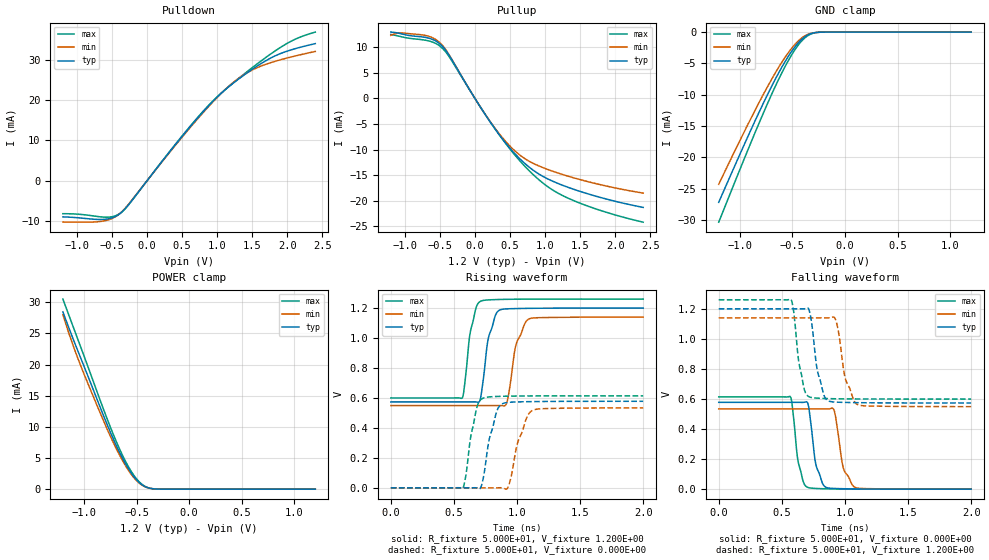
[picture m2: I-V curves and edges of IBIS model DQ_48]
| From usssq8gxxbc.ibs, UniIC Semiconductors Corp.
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|   Model DQ_48
[Model] DQ_48
Model_type I/O
Polarity   Non-Inverting
Enable   Active-High
Vinl =  8.300E-01
Vinh =  9.700E-01
Vmeas =  8.400E-01
Rref =  5.000E+01
Vref =  1.200E+00
C_comp   6.590E-13   6.530E-13   6.678E-13
C_comp_pullup   3.168E-13   3.162E-13   3.180E-13
C_comp_pulldown   3.268E-13   3.197E-13   3.362E-13
[Model Spec]
Vinh   9.700E-01   9.250E-01   1.015E+00
Vinl   8.300E-01   7.850E-01   8.750E-01
Vmeas   8.400E-01   7.980E-01   8.820E-01
Vref   1.200E+00   1.140E+00   1.260E+00
Rref   5.000E+01   5.000E+01   5.000E+01
[Temperature Range]   4.500E+01   9.500E+01   0.000E+00
[Voltage Range]   1.200E+00   1.140E+00   1.260E+00
[C Comp Corner]
C_comp_pullup   3.168E-13   3.180E-13   3.162E-13
C_comp_pulldown   3.268E-13   3.197E-13   3.362E-13
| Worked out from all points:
|   slope of the pulldown table from 0 to 0.18 V, typ, clamps not added: 44.6 ohm
|   slope of the pullup table from 0 to 0.18 V, typ, clamps not added: 46.9 ohm
|   GND clamp passes 1 mA (typ) near -0.40 V on its own axis
|   POWER clamp passes 1 mA (typ) near -0.47 V on its own axis
|   rising waveform, R_fixture 5.000E+01, V_fixture 1.200E+00: 20-80 % time 74.8ps typ, 87.1ps min, 65.1ps max; typ from 0.574 V to 1.2 V
|   rising waveform, R_fixture 5.000E+01, V_fixture 0.000E+00: 20-80 % time 80.7ps typ, 98.7ps min, 68.3ps max; typ from 0 V to 0.578 V
|   falling waveform, R_fixture 5.000E+01, V_fixture 0.000E+00: 20-80 % time 64.2ps typ, 69.4ps min, 57.5ps max; typ from 0.578 V to 0 V
|   falling waveform, R_fixture 5.000E+01, V_fixture 1.200E+00: 20-80 % time 70.3ps typ, 85.6ps min, 60.9ps max; typ from 1.2 V to 0.574 V
[Pulldown]
|Voltage   I(typ)   I(min)   I(max)
-1.2V     -8.95mA    -10.23mA   -8.16mA
-645mV    -9.589mA   -10.04mA   -8.974mA
-497mV    -9.184mA   -9.333mA   -8.904mA
-386mV    -8.143mA   -8.108mA   -8.086mA
-275mV    -6.168mA   -6.062mA   -6.22mA
687mV     14.86mA    14.65mA    15mA
983mV     20.46mA    20.34mA    20.53mA
1.205V    23.86mA    24.02mA    23.93mA
1.464V    27.19mA    27.13mA    27.55mA
1.797V    30.71mA    29.46mA    31.83mA
2.093V    32.65mA    30.85mA    34.92mA
2.4V      34mA       32.06mA    36.86mA
[Pullup]
|Voltage   I(typ)   I(min)   I(max)
-1.2V     12.95mA    12.32mA    12.49mA
-1.041V   12.59mA    12.78mA    12.02mA
-745mV    12mA       12.39mA    11.45mA
-486mV    10.48mA    10.69mA    10.06mA
-375mV    8.569mA    8.662mA    8.299mA
32mV      -704.1uA   -701.9uA   -692.2uA
291mV     -6.036mA   -5.916mA   -6.023mA
513mV     -9.935mA   -9.504mA   -10.11mA
735mV     -12.98mA   -11.95mA   -13.58mA
1.031V    -15.66mA   -13.83mA   -17.16mA
1.327V    -17.35mA   -15.18mA   -19.47mA
2.4V      -21.28mA   -18.49mA   -24.17mA
[GND_clamp]
|Voltage   I(typ)   I(min)   I(max)
-1.2V     -27.2mA    -24.33mA   -30.38mA
-875mV    -14.93mA   -13.17mA   -16.89mA
-750mV    -10.47mA   -9.157mA   -11.95mA
-650mV    -7.145mA   -6.184mA   -8.244mA
-575mV    -4.884mA   -4.175mA   -5.699mA
-500mV    -2.92mA    -2.45mA    -3.459mA
-425mV    -1.383mA   -1.13mA    -1.679mA
-375mV    -673.2uA   -542.8uA   -837uA
-300mV    -135.5uA   -116.3uA   -166.1uA
-225mV    -14.67uA   -15.93uA   -14.24uA
1.2V      0A         0A         0A
[POWER_clamp]
|Voltage   I(typ)   I(min)   I(max)
-1.2V     28.45mA    28mA       30.5mA
-1.125V   25.07mA    24.12mA    27.08mA
-1.025V   20.8mA     19.57mA    22.55mA
-850mV    13.34mA    12.42mA    14.46mA
-750mV    9.2mA      8.545mA    10.01mA
-650mV    5.523mA    5.115mA    6.037mA
-575mV    3.235mA    2.981mA    3.547mA
-500mV    1.501mA    1.371mA    1.657mA
-450mV    723.1uA    662.7uA    804.4uA
-375mV    148.3uA    148.7uA    156.1uA
-300mV    17.6uA     22.56uA    14.19uA
1.2V      0A         0A         0A
[Ramp]
| variable   typ   min   max
dV/dt_r   3.466E-01/8.120E-11   3.202E-01/9.979E-11   3.683E-01/6.823E-11
dV/dt_f   3.759E-01/7.046E-11   3.546E-01/8.551E-11   3.962E-01/6.107E-11
R_load = 5.000E+01
[Rising Waveform]
R_fixture= 5.000E+01
V_fixture= 1.200E+00
V_fixture_min= 1.140E+00
V_fixture_max= 1.260E+00
|time   V(typ)   V(min)   V(max)
0s        573.5mV    548.8mV    599.7mV
565ps     573.6mV    548.8mV    598.5mV
632ps     573.7mV    548.8mV    1.049V
712ps     603.2mV    548.9mV    1.246V
770ps     987.6mV    548.9mV    1.254V
856ps     1.184V     549.2mV    1.257V
916ps     1.194V     561.6mV    1.258V
986ps     1.196V     934.4mV    1.259V
1.086ns   1.198V     1.123V     1.259V
2ns       1.2V       1.14V      1.26V
[Rising Waveform]
R_fixture= 5.000E+01
V_fixture= 0.000E+00
V_fixture_min= 0.000E+00
V_fixture_max= 0.000E+00
|time   V(typ)   V(min)   V(max)
0s        212nV      624.9nV    103.2nV
571ps     74.47uV    23.77uV    -2.692mV
677ps     -125.2uV   66.44uV    521mV
740ps     99.55mV    55.33uV    601.2mV
788ps     351.8mV    73.19uV    607.5mV
884ps     561.1mV    -314.5uV   611mV
934ps     570.6mV    14.74mV    611.9mV
1.005ns   573.5mV    301.9mV    612.7mV
1.115ns   575.4mV    513.1mV    613.4mV
2ns       577.6mV    533.7mV    613.8mV
[Falling Waveform]
R_fixture= 5.000E+01
V_fixture= 0.000E+00
V_fixture_min= 0.000E+00
V_fixture_max= 0.000E+00
|time   V(typ)   V(min)   V(max)
0s        577.7mV    533.9mV    613.8mV
565ps     577.6mV    533.9mV    617.4mV
632ps     577.6mV    533.9mV    172.4mV
705ps     573.2mV    533.9mV    11.81mV
770ps     163.5mV    533.9mV    4.705mV
846ps     14.02mV    533.5mV    2.506mV
916ps     4.591mV    520.9mV    1.432mV
987ps     2.974mV    141.6mV    820uV
1.078ns   1.762mV    12.84mV    406.4uV
2ns       13.41uV    118.4uV    1.177uV
[Falling Waveform]
R_fixture= 5.000E+01
V_fixture= 1.200E+00
V_fixture_min= 1.140E+00
V_fixture_max= 1.260E+00
|time   V(typ)   V(min)   V(max)
0s        1.2V       1.14V      1.26V
572ps     1.2V       1.14V      1.263V
640ps     1.2V       1.14V      820.1mV
717ps     1.189V     1.14V      614.1mV
781ps     791.1mV    1.14V      605.5mV
864ps     589.4mV    1.14V      602.6mV
927ps     579.4mV    1.125V     601.5mV
1.006ns   577.1mV    727.5mV    600.7mV
1.097ns   575.6mV    563.9mV    600.2mV
2ns       573.5mV    548.9mV    599.7mV
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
